PROGRAM MAIN
VAR
	ToPC1 AT %Q*:ARRAY[0..127] OF BYTE;
	fbTON1: TON;
	q1: BOOL;
	FromPC1 AT %I*:ARRAY[0..127] OF BYTE;	//接收的数据
	fbTON2: TON;
	fbTON3: TON;
	ComError: BOOL;	// 通信错误
END_VAR

fbTON1(IN:=NOT fbTON1.Q , PT:=T#500MS , Q=> , ET=> );
IF fbTON1.Q THEN
	q1:=NOT q1;
END_IF
ToPC1[0].0:=q1;

//心跳检测
fbTON2(IN:=NOT FromPC1[0].0 , PT:=T#1S , Q=> , ET=> );
fbTON3(IN:=FromPC1[0].0 , PT:=T#1S , Q=> , ET=> );
IF fbTON2.Q OR fbTON3.Q THEN
	ComError:=TRUE;
ELSE
	ComError:=FALSE;
END_IF

END_PROGRAM
